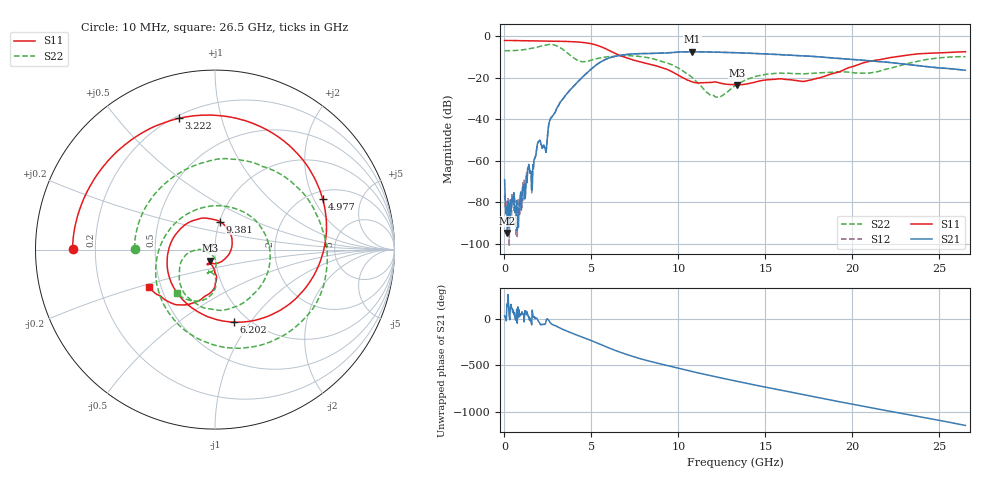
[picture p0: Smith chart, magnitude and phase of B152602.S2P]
!  2-Port S-parameters saved by WinCal
! VAR MeasName=S-Parameters (CALIBRATED_DATA) read from VNA (N5242A)
! VAR MeasDate=2016-1-5 16:25:04
! VAR NAME=B152602
! VAR FILENAME=B152602.S2P
! VAR DATE=2016-1-5 16:25:04
! VAR PHYS_PORTS=1,2
# Hz S DB R 50
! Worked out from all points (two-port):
!   801 points, 10 MHz to 26.5 GHz, reference 50 ohm
!   highest |S21| = -7.45 dB at 10.8 GHz (marker M1); lowest = -94.9 dB at 175.6 MHz (marker M2)
!   |S21| within 3 dB of the highest: 6.005 GHz to 18.87 GHz (12.86 GHz wide, 103 % of centre)
!   lowest |S11| = -23.5 dB at 13.39 GHz (marker M3), VSWR 1.14, Z = 47.1 - j5.86 ohm
!   |S11| at or under -10 dB: 6.888 GHz to 22.42 GHz (15.53 GHz wide, 106 % of centre)
!   |S22| runs from -29.4 to -3.9 dB; largest |S21 - S12| = 0.0024
!   S11 on the Smith chart (normalised r, x): 10 MHz: 0.12, +0.00; 3.222 GHz: 0.21, +0.74; 4.977 GHz: 2.33, +2.35; 6.202 GHz: 0.86, -0.84; 9.381 GHz: 1.01, +0.32; 26.5 GHz: 0.43, -0.22
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1e7  -2.01 179.8  -69.18 29.9  -76.40 67.0  -6.97 179.3
1.755625e8  -2.01 176.4  -94.87 130.6  -82.73 -159.7  -6.95 169.2
8.70925e8  -2.10 162.1  -79.58 22.2  -86.49 14.8  -6.70 126.0
1.533175e9  -2.17 148.3  -65.82 -33.6  -66.69 -46.3  -5.83 80.6
1.963638e9  -2.22 138.8  -50.83 -32.4  -50.67 -33.2  -5.03 47.2
2.427212e9  -2.28 127.7  -52.85 -9.2  -52.95 -10.5  -4.16 3.6
3.221912e9  -2.40 105.5  -31.62 -103.4  -31.66 -103.5  -5.56 -92.1
3.751712e9  -2.54 87.3  -26.09 -146.5  -26.11 -146.6  -8.95 -157.7
4.447075e9  -2.91 56.5  -20.01 163.8  -20.02 163.9  -12.21 112.7
4.976875e9  -3.57 25.3  -15.88 126.1  -15.88 126.2  -11.55 51.3
6.202038e9  -7.57 -75.3  -9.96 31.3  -9.95 31.3  -9.74 -39.6
7.1623e9  -10.79 -155.8  -8.65 -32.1  -8.64 -32.2  -9.36 -81.1
8.851038e9  -14.56 110.1  -8.14 -119.9  -8.15 -120.1  -11.60 -139.0
9.380838e9  -16.00 79.7  -8.00 -143.3  -8.01 -143.3  -13.03 -152.0
1.080468e10  -22.01 -25.1  -7.45 153.0  -7.45 153.0  -19.95 -180.0
1.222851e10  -22.18 -100.4  -7.68 93.7  -7.68 93.8  -29.35 -128.6
1.3255e10  -23.36 -112.7  -7.91 53.1  -7.91 52.9  -23.83 -86.8
1.338745e10  -23.48 -112.6  -7.93 47.8  -7.95 47.9  -23.21 -85.7
1.514241e10  -20.96 -112.6  -8.57 -19.0  -8.58 -19.1  -18.21 -98.2
1.769208e10  -20.89 -100.3  -9.69 -113.4  -9.67 -113.3  -17.84 -105.7
2.209604e10  -10.42 -107.9  -12.62 89.7  -12.56 89.5  -15.57 -88.7
2.65e10  -7.43 -150.3  -16.37 -63.9  -16.36 -64.4  -9.86 -130.9
